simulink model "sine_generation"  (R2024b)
settings: Solver=VariableStepAuto  StartTime=0.0  StopTime=10.0  RelTol=1e-3
undefined symbols (not defined in the file): f, fs
libraries: hdlsllib x2

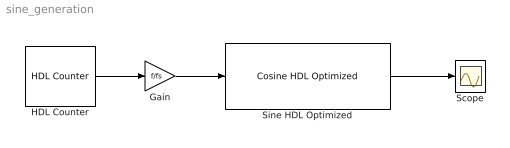
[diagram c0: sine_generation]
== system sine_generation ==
  Gain : Gain  Gain=f/fs
  HDL Counter : hdlsllib/Sources/HDL Counter  CountType=Modulo  CountInit=0  CountStep=1  CountMax=fs  CountFromType=Specify  CountFrom=0  CountResetPort=off  CountLoadPort=off  CountEnbPort=off  CountDirPort=off  CountHitOutputPort=off  CountDataType=Signed  CountWordLen=32  CountFracLen=0  CountSampTime=1/fs
  Scope : Scope
  Sine HDL Optimized : hdlsllib/Lookup Tables/Cosine HDL Optimized  OutputFormula=sin(2*pi*u)  NumDataPoints=128  TableDataTypeStr=fixdt(0,16,15)  SimulateLUTROMDelay=off
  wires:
  HDL Counter/1 -> Gain/1
  Sine HDL Optimized/1 -> Scope/1
  Gain/1 -> Sine HDL Optimized/1
